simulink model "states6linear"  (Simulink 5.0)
settings: Solver=ode45  StartTime=0.0  StopTime=10  MaxStep=1e-3  RelTol=1e-3
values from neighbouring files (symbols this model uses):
  alpha0 = 3.77    [Load_Parameters.m]
  ap = -2.3    [Load_Parameters.m]
  B = 0.016033    [Load_Parameters.m]
  bp = 15369    [Load_Parameters.m]
  Gmp = 4.5e-9    (= 4.5e-09)    [Load_Parameters.m]
  Mo = -2.08e-5    (= -2.08e-05)    [Load_Parameters.m]
  n0 = 800    [Load_Parameters.m]
  p0 = 24873    [Load_Parameters.m]
  T_p = 20    [Load_Parameters.m]
libraries: simulink_extras x1

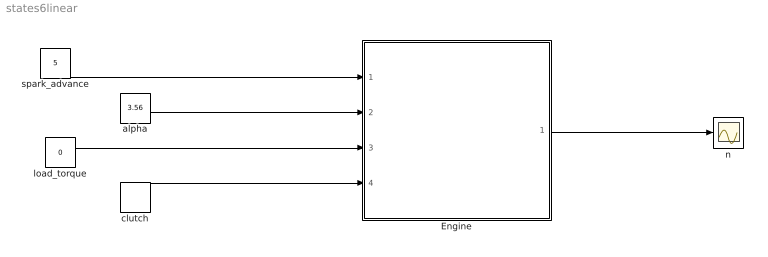
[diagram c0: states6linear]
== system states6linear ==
  Engine : Subsystem
  alpha : Constant  Value=3.56
  clutch : DiscretePulseGenerator  PulseType=Time based  Period=.4  PulseWidth=50
  load_torque : Constant  Value=0
  n : Scope
  spark_advance : Constant  Value=5
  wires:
  spark_advance/1 -> Engine/1(In1)
  alpha/1 -> Engine/2(alpha)
  load_torque/1 -> Engine/3(load_torque1)
  clutch/1 -> Engine/4(clutch)
  Engine/1(Out1) -> n/1

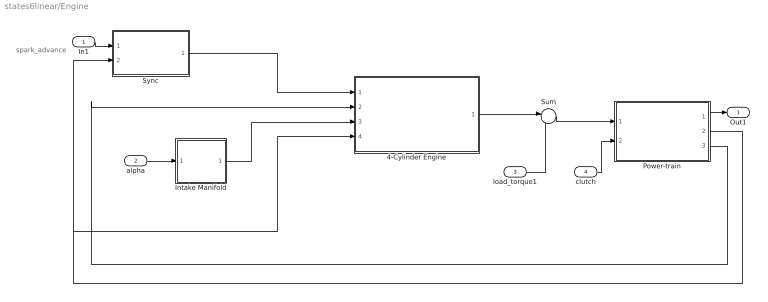
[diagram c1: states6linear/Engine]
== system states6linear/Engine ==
  note: spark_advance
  In1 : Inport
  alpha : Inport  Port=2
  load_torque1 : Inport  Port=3
  clutch : Inport  Port=4
  4-Cylinder Engine : Subsystem
  Intake Manifold : Subsystem
  Power-train : Subsystem
  Sum : Sum  Inputs=|+-
  Sync : Subsystem
  Out1 : Outport
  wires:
  4-Cylinder Engine/1(T) -> Sum/1
  Power-train/2(theta) -> Sync/2(theta), 4-Cylinder Engine/4(theta)
  Sum/1 -> Power-train/1(T_eff)
  Sync/1(spark) -> 4-Cylinder Engine/1(spark)
  Power-train/3(DC) -> 4-Cylinder Engine/2(DC)
  Intake Manifold/1(m) -> 4-Cylinder Engine/3(m)
  load_torque1/1 -> Sum/2
  alpha/1 -> Intake Manifold/1(alpha)
  clutch/1 -> Power-train/2(clutch)
  In1/1 -> Sync/1(spark_advance)
  Power-train/1(n) -> Out1/1

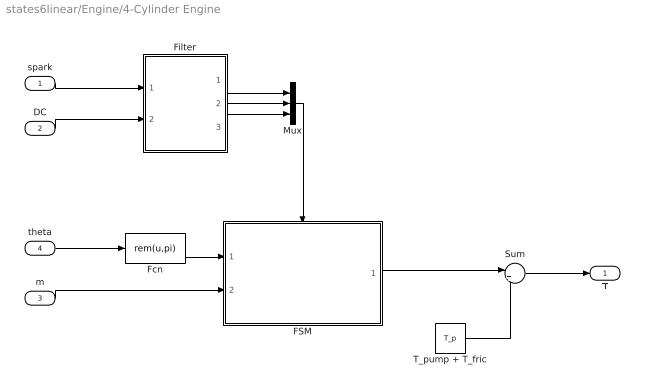
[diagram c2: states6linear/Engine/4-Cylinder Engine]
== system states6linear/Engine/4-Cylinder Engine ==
  spark : Inport
  DC : Inport  Port=2
  m : Inport  Port=3
  theta : Inport  Port=4
  FSM : Stateflow chart  TreatAsAtomicUnit=on
  Fcn : Fcn  Expr=rem(u,pi)
  Filter : Subsystem
  Mux : Mux  Inputs=3
  Sum : Sum  Inputs=|+-
  T_pump + T_fric : Constant  Value=T_p
  T : Outport
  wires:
  Mux/1 -> FSM/Trigger
  Filter/2(DC) -> Mux/2
  Filter/3(sparkDC) -> Mux/3
  Filter/1(spark) -> Mux/1
  theta/1 -> Fcn/1
  DC/1 -> Filter/2(DC_in)
  spark/1 -> Filter/1(spark_in)
  Fcn/1 -> FSM/1(theta)
  m/1 -> FSM/2(mc)
  Sum/1 -> T/1
  FSM/1(T_eff) -> Sum/1
  T_pump + T_fric/1 -> Sum/2

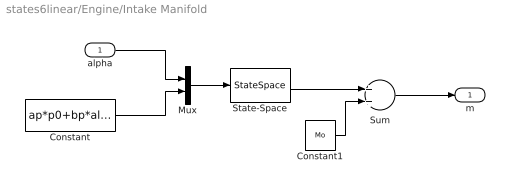
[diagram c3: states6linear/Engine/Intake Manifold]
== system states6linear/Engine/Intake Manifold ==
  alpha : Inport
  Constant : Constant  Value=ap*p0+bp*alpha0
  Constant1 : Constant  Value=Mo
  Mux : Mux  Inputs=2
  State-Space : StateSpace  A=ap  B=[bp -1]  C=Gmp  D=[0 0]  X0=p0
  Sum : Sum
  m : Outport
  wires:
  State-Space/1 -> Sum/1
  Mux/1 -> State-Space/1
  alpha/1 -> Mux/1
  Constant/1 -> Mux/2
  Sum/1 -> m/1
  Constant1/1 -> Sum/2

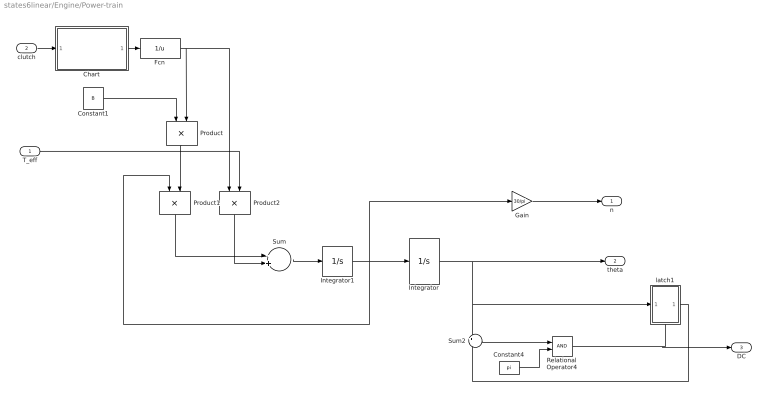
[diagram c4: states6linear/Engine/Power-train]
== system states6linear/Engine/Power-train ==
  T_eff : Inport
  clutch : Inport  Port=2
  Chart : Stateflow chart
  Constant1 : Constant  Value=B
  Constant4 : Constant  Value=pi
  Fcn : Fcn  Expr=1/u
  Gain : Gain  Gain=30/pi
  Integrator : Integrator
  Integrator1 : Integrator  InitialCondition=pi*n0/30
  Product : Product  Orientation=down
  Product1 : Product  Orientation=down
  Product2 : Product  Orientation=down
  Relational Operator4 : RelationalOperator
  Sum : Sum  Inputs=-+
  Sum2 : Sum  Inputs=+-
  latch1 : Subsystem  TreatAsAtomicUnit=on
  n : Outport
  theta : Outport  Port=2
  DC : Outport  Port=3
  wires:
  T_eff/1 -> Product2/2
  Integrator/1 -> theta/1, latch1/1(In), Sum2/1
  latch1/1(Out) -> Sum2/2
  Sum2/1 -> Relational Operator4/1
  Constant4/1 -> Relational Operator4/2
  Relational Operator4/1 -> latch1/Trigger, DC/1
  Chart/1(Jx) -> Fcn/1
  Constant1/1 -> Product/1
  Fcn/1 -> Product/2, Product2/1
  Product/1 -> Product1/2
  Product1/1 -> Sum/1
  Product2/1 -> Sum/2
  Sum/1 -> Integrator1/1
  Integrator1/1 -> Product1/1, Integrator/1, Gain/1
  clutch/1 -> Chart/1(clutch)
  Gain/1 -> n/1

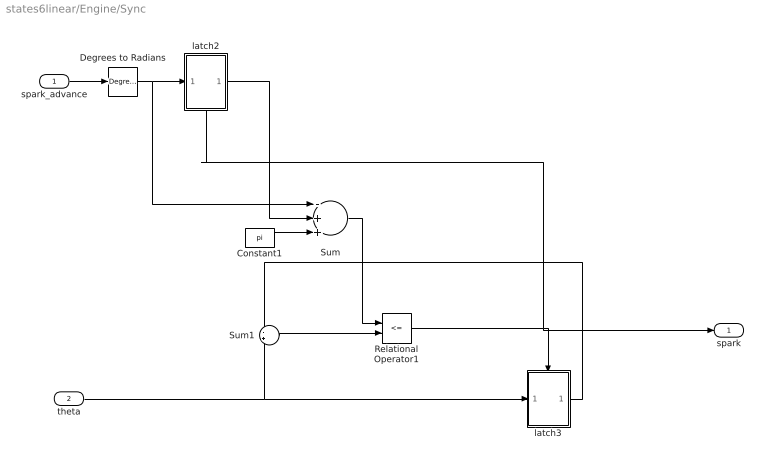
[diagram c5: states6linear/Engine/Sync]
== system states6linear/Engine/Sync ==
  spark_advance : Inport
  theta : Inport  Port=2
  Constant1 : Constant  Value=pi
  Degrees to Radians : simulink_extras/Transformations/Degrees to Radians
  Relational Operator1 : RelationalOperator  Operator=<=
  Sum : Sum  Inputs=-++
  Sum1 : Sum  Inputs=-+
  latch2 : Subsystem  TreatAsAtomicUnit=on
  latch3 : Subsystem  TreatAsAtomicUnit=on
  spark : Outport
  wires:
  latch2/1(Out) -> Sum/2
  Relational Operator1/1 -> latch3/Trigger, latch2/Trigger, spark/1
  Sum1/1 -> Relational Operator1/2
  latch3/1(Out) -> Sum1/1
  Sum/1 -> Relational Operator1/1
  Constant1/1 -> Sum/3
  theta/1 -> latch3/1(In), Sum1/2
  Degrees to Radians/1 -> latch2/1(In), Sum/1
  spark_advance/1 -> Degrees to Radians/1

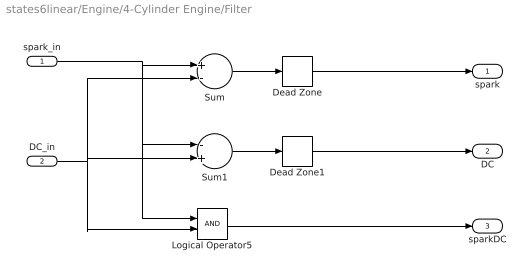
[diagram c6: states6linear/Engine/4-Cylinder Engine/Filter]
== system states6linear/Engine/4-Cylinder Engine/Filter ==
  spark_in : Inport
  DC_in : Inport  Port=2
  Dead Zone : DeadZone  LowerValue=-2  UpperValue=0
  Dead Zone1 : DeadZone  LowerValue=-2  UpperValue=0
  Logical Operator5 : Logic
  Sum : Sum  Inputs=+-
  Sum1 : Sum  Inputs=-+
  spark : Outport
  DC : Outport  Port=2
  sparkDC : Outport  Port=3
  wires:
  DC_in/1 -> Sum/2, Sum1/2, Logical Operator5/2
  Sum/1 -> Dead Zone/1
  Sum1/1 -> Dead Zone1/1
  spark_in/1 -> Sum/1, Sum1/1, Logical Operator5/1
  Dead Zone1/1 -> DC/1
  Dead Zone/1 -> spark/1
  Logical Operator5/1 -> sparkDC/1

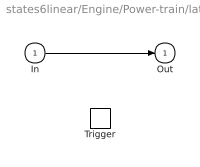
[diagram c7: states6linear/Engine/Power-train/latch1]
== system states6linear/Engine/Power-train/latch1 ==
  In : Inport
  Trigger : TriggerPort
  Out : Outport  InitialOutput=0
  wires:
  In/1 -> Out/1

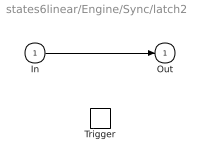
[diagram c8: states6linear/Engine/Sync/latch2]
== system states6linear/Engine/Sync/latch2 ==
  In : Inport
  Trigger : TriggerPort
  Out : Outport  InitialOutput=0
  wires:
  In/1 -> Out/1

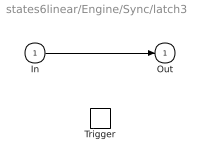
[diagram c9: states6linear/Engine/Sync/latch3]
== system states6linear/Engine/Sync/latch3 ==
  In : Inport
  Trigger : TriggerPort
  Out : Outport  InitialOutput=0
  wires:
  In/1 -> Out/1

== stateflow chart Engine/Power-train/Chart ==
  state Clutch_closed/
    entry: Jx =Jc;
  state Clutch_open/
    entry: Jx =Jo;
  Clutch_closed -> Clutch_open : [clutch]
  Clutch_open -> Clutch_closed : [~clutch]
  (default) -> Clutch_closed

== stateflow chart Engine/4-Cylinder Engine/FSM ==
  state Sl_minus
  state Sl
  state Sl_plus
  state eff = eta(ang) [function]
    (default) -> (junction 18) : {eff = eta_a+sqrt(eta_b+eta_c*ang);}
  Sl -> Sl_minus : dc/{me = mc;T_eff=0;}
  Sl_minus -> Sl : spark/{T_eff = (G*me+T0)*eta(-theta);}
  Sl -> Sl_plus : spark/{fi = pi-theta;}
  Sl_plus -> Sl : dc/{T_eff = (G*mc+T0)*eta(fi);}
  Sl -> Sl : sparkdc/{T_eff = (G*mc+T0)*eta(0);}
  (default) -> Sl
